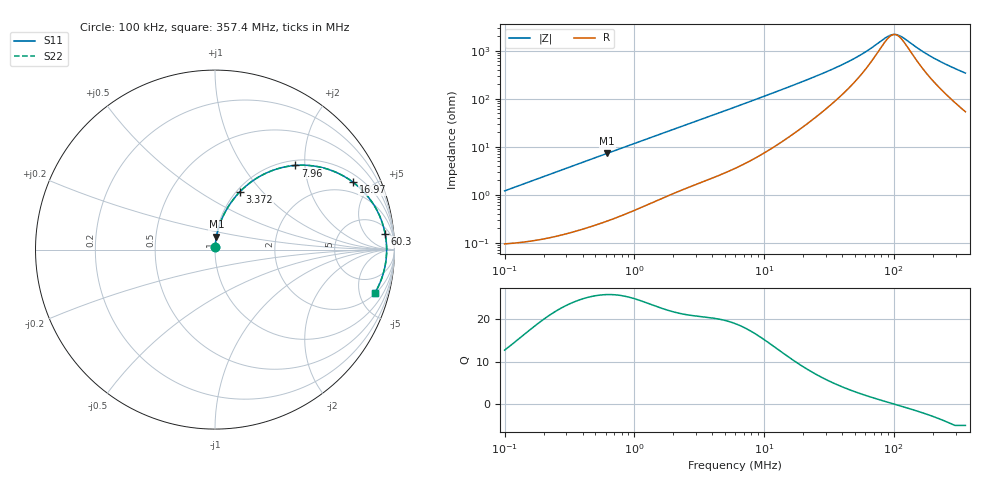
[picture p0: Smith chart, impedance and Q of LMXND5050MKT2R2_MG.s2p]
! LMXND5050MKT2R2_MG  S-PARAMETER MODEL  ( General Type )
! Model Generated by TAIYO YUDEN Corporation (http://www.ty-top.com)
! Version 1.0
! TAIYO YUDEN Control No. 191023NI43SB-FBB
! Copyright(c) 2019 TAIYO YUDEN CO.,LTD. All Rights Reserved.
! Product Description (link to TY-COMPAS)
! https://ds.yuden.co.jp/TYCOMPAS/or/detail?pn=LMXND5050MKT2R2MMG&u=M
! Products Name : Inductors
! Characteristics :
!  Inductance : 2.2 uH , SRF(min) : 70 MHz , DC Resistance(max) : 0.102 Ohm
!  Rated Current : Saturation :3100 mA , Temp Rise : 2000 mA
!  Case Size : 4.9 x 4.9 / 0.193 x 0.193 [mm/inch] , Thickness : 1.2 / 0.047 [mm/inch]
!  (Conditions: Temperature = 25 degC , DC Bias Current/Voltage = 0A / 0V)
! External Node Assignments :
!  1  o---GGG---o  2
! GND o---------o GND
! Frequency Range : 0.1MHz  -  357.398349MHz  [ 402 STEP ]
# MHz S RI R 50
! Freq[MHz].  S11 Real  S11 Imag  S21 Real  S21 Imag  S12 Real  S12 Imag  S22 Real  S22 Imag
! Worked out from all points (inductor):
!   401 points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, 100 kHz to 357.4 MHz, reference 50 ohm
!   read as one part in series: L = 1.92 uH near 104.2 kHz
!   highest Q = 25.8 at 617.4 kHz (marker M1), where L = 1.88 uH
!   self-resonance near 101.3 MHz
!   S11 on the Smith chart (normalised r, x): 100 kHz: 1.00, +0.02; 3.372 MHz: 1.04, +0.77; 7.96 MHz: 1.10, +1.79; 16.97 MHz: 1.38, +3.86; 60.3 MHz: 9, +17; 357.4 MHz: 2.08, -6.80
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0.1  0.00109 0.012  0.9989 -0.012  0.9989 -0.012  0.00109 0.012
0.393689  0.00408 0.0466  0.9959 -0.0466  0.9959 -0.0466  0.00408 0.0466
0.617414  0.00809 0.0722  0.9919 -0.0722  0.9919 -0.0722  0.00809 0.0722
1.549909  0.0385 0.1716  0.9615 -0.1716  0.9615 -0.1716  0.0385 0.1716
2.381478  0.0796 0.2482  0.9204 -0.2482  0.9204 -0.2482  0.0796 0.2482
3.371752  0.1399 0.3234  0.8601 -0.3234  0.8601 -0.3234  0.1399 0.3234
4.489686  0.2164 0.3875  0.7836 -0.3875  0.7836 -0.3875  0.2164 0.3875
6.101817  0.3294 0.4442  0.6706 -0.4442  0.6706 -0.4442  0.3294 0.4442
7.960432  0.4485 0.469  0.5515 -0.469  0.5515 -0.469  0.4485 0.469
11.27056  0.6108 0.4534  0.3892 -0.4534  0.3892 -0.4534  0.6108 0.4534
16.96693  0.7689 0.3756  0.2311 -0.3756  0.2311 -0.3756  0.7689 0.3756
23.53582  0.8535 0.2933  0.1465 -0.2933  0.1465 -0.2933  0.8535 0.2933
40.05754  0.9256 0.167  0.0744 -0.167  0.0744 -0.167  0.9256 0.167
60.30341  0.9482 0.087  0.0518 -0.087  0.0518 -0.087  0.9482 0.087
85.37896  0.9556 0.0278  0.0444 -0.0278  0.0444 -0.0278  0.9556 0.0278
92.65788  0.9562 0.0145  0.0438 -0.0145  0.0438 -0.0145  0.9562 0.0145
100.5574  0.9564 0.00122  0.0436 -0.00122  0.0436 -0.00122  0.9564 0.00122
111.3854  0.9562 -0.0154  0.0438 0.0154  0.0438 0.0154  0.9562 -0.0154
164.2869  0.9496 -0.0807  0.0504 0.0807  0.0504 0.0807  0.9496 -0.0807
197.4918  0.9426 -0.1146  0.0574 0.1146  0.0574 0.1146  0.9426 -0.1146
268.406  0.9224 -0.1773  0.0776 0.1773  0.0776 0.1773  0.9224 -0.1773
357.3983  0.8894 -0.2442  0.1106 0.2442  0.1106 0.2442  0.8894 -0.2442
